(* Logix 5000 AddOnInstructionDefinition export SetupSignVariables; software revision 17.00 *)

ADD_ON_INSTRUCTION SetupSignVariables   (* revision 1.0, vendor Electronic Displays, Inc., ExecuteEnableInFalse *)
// Setup to
// Four Variables
// to LED Sign
// Revision note:
// Original Release
// 11-01-2012
// c.elston
VAR_IN_OUT
   Address : STRING; {required}   // "00" = all signs "01" = address 01 "02" = address 02 etc...(see protocol)
   FileLabel : STRING; {required}   // "A" = default etc...(see protocol)
END_VAR
VAR_INPUT
   ENVariable1Message : BOOL; {visible}   // 0 = don't setup variable 1 = setup variable
END_VAR
VAR_IN_OUT
   Variable1Name : STRING; {required}   // Name of variable Default is = U
END_VAR
VAR_INPUT
   ENVariable2Message : BOOL; {visible}   // 0 = don't setup variable 1 = setup variable
END_VAR
VAR_IN_OUT
   Variable2Name : STRING; {required}   // Name of variable Default is = V
END_VAR
VAR_INPUT
   ENVariable3Message : BOOL; {visible}   // 0 = don't setup variable 1 = setup variable
END_VAR
VAR_IN_OUT
   Variable3Name : STRING; {required}   // Name of variable Default is = W
END_VAR
VAR_INPUT
   ENVariable4Message : BOOL; {visible}   // 0 = don't setup variable 1 = setup variable
END_VAR
VAR_IN_OUT
   Variable4Name : STRING; {required}   // Name of variable Default is = X
END_VAR
VAR_OUTPUT
   EN : BOOL; {visible}   // Instruction Interface Enable Bit
   DN : BOOL; {visible}   // Instruction Interface Done Bit
   ER : BOOL; {visible}   // Instruction Interface Error Bit
   IP : BOOL; {visible}   // Instruction Interface InProcess Bit
END_VAR
VAR_IN_OUT
   map_SignInput : SINT[32]; {required}   // Ethernet/IP LEDSIGN.I Data I/O Mapping
   map_SignOutput : SINT[496]; {required}   // Ethernet/IP LEDSIGN.O Data I/O Mapping
   Packet1Sent : STRING; {required}   // The actual packet sent to the sign (Packet1)
   Packet2Sent : STRING; {required}   // The actual packet sent to the sign (Packet2)
   Packet3Sent : STRING; {required}   // The actual packet sent to the sign (Packet3)
END_VAR
VAR
   SEQ : DINT;   // Sequence Number
   OktoCycle : BOOL;   // Ok to Cycle
   InCycle : BOOL;   // Incycle
   Error : BOOL;   // Error
   Enabled : BOOL;   // Enable ON Bit
   Done : BOOL;   // Done
   Disabled : BOOL;   // Disabled OFF Bit
   SignETX : STRING := '^C';   // DO NOT EDIT = ^C
   SignFileLabel : STRING;
   SignSOH : STRING := '^A';   // DO NOT EDIT = ^A
   SignAddress : STRING;
   SignSTX : STRING := '^B';   // DO NOT EDIT = ^B
   SignNULL : STRING;
   SignVariable4 : STRING;
   SignVariable3 : STRING;
   SignVariable2 : STRING;
   SignVariable1 : STRING;
   SignSetMemoryCommand : STRING := 'SM';   // DO NOT EDIT = SM
   SignCommandCode : STRING := 'C';   // DO NOT EDIT = C
   SignSizeVariableCommand : STRING := '0010';   // DO NOT EDIT = 0010 (16 bytes of memory) enough for 16 characters
   SignFileVariableCommand : STRING := 'V';   // DO NOT EDIT = V
   TotalPacketCount : DINT[7];   // Total Character Count
   Select : DINT;   // Packet Array Select
   PacketMax : DINT := 82;   // Max Packet Count
   PacketCount : DINT[7];
   Packet6Offset : DINT;
   Packet5Offset : DINT;
   Packet4Offset : DINT;
   Packet3Offset : DINT;
   Packet2Offset : DINT;
   Packet1Offset : DINT;
   Packet : STRING[7];   // Packet Array to send to sign
END_VAR

ROUTINE EnableInFalse   (* ladder *)
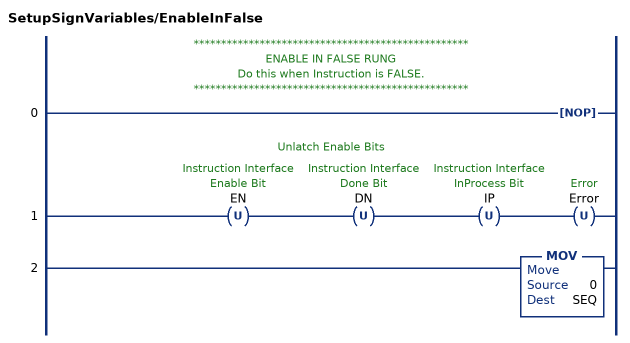
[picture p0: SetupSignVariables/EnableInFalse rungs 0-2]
   // **************************************************
   // ENABLE IN FALSE RUNG
   // Do this when Instruction is FALSE.
   // **************************************************
   0: NOP();
   // Unlatch Enable Bits
   1: OTU(EN)OTU(DN)OTU(IP)OTU(Error);
   2: MOV(0,SEQ);
END_ROUTINE

ROUTINE Logic   (* ladder *)
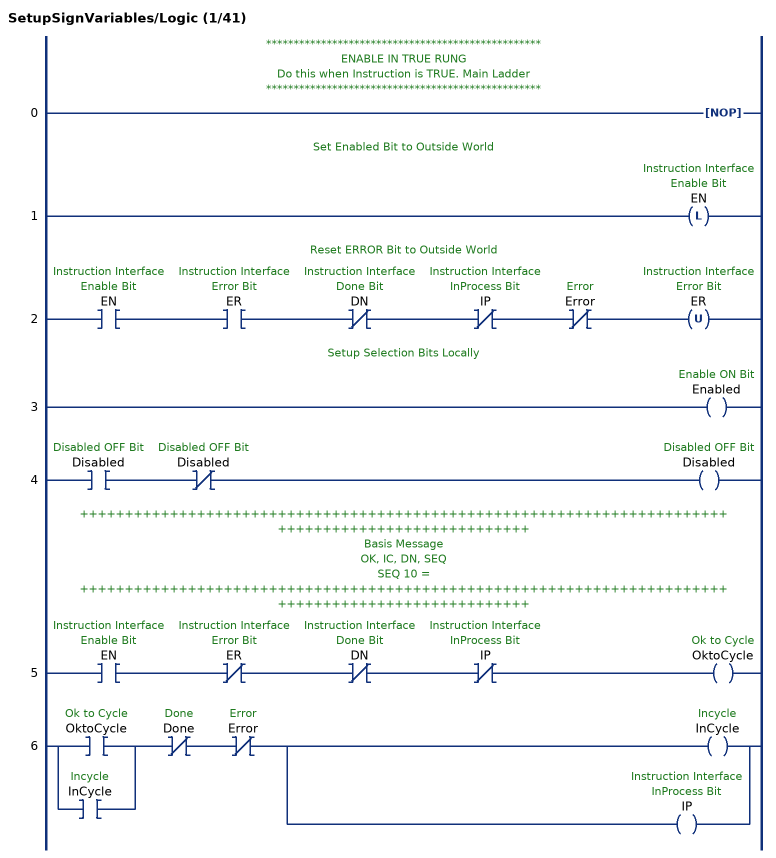
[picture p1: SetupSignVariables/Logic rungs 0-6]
   // **************************************************
   // ENABLE IN TRUE RUNG
   // Do this when Instruction is TRUE. Main Ladder
   // **************************************************
   0: NOP();
   // Set Enabled Bit to Outside World
   1: OTL(EN);
   // Reset ERROR Bit to Outside World
   2: XIC(EN)XIC(ER)XIO(DN)XIO(IP)XIO(Error)OTU(ER);
   // Setup Selection Bits Locally
   3: OTE(Enabled);
   4: XIC(Disabled)XIO(Disabled)OTE(Disabled);
   // ++++++++++++++++++++++++++++++++++++++++++++++++++++++++++++++++++++++++++++++++++++++++++++++++++++
   // Basis Message
   // OK, IC, DN, SEQ
   // SEQ 10 =
   // ++++++++++++++++++++++++++++++++++++++++++++++++++++++++++++++++++++++++++++++++++++++++++++++++++++
   5: XIC(EN)XIO(ER)XIO(DN)XIO(IP)OTE(OktoCycle);
   6: [XIC(OktoCycle) ,XIC(InCycle) ]XIO(Done)XIO(Error)[OTE(InCycle) ,OTE(IP) ];
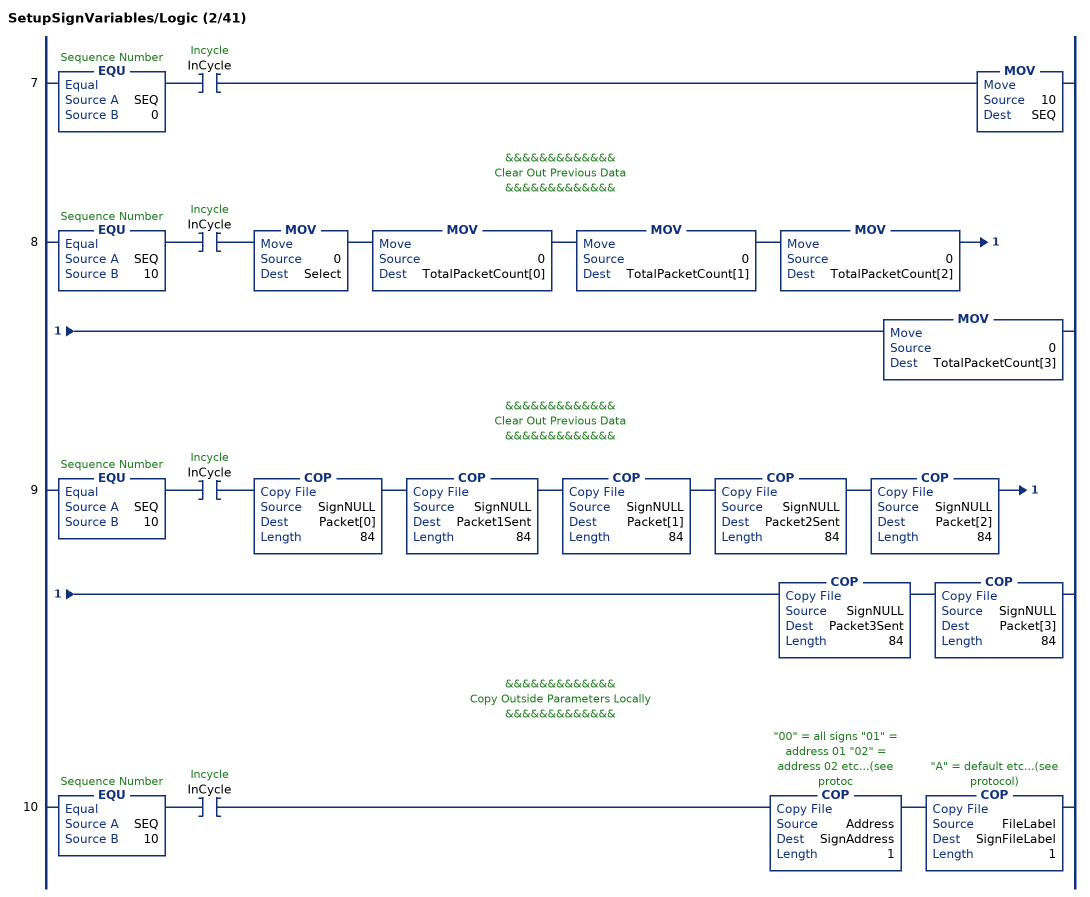
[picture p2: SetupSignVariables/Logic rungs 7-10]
   7: EQU(SEQ,0)XIC(InCycle)MOV(10,SEQ);
   // &&&&&&&&&&&&&
   // Clear Out Previous Data
   // &&&&&&&&&&&&&
   8: EQU(SEQ,10)XIC(InCycle)MOV(0,Select)MOV(0,TotalPacketCount[0])MOV(0,TotalPacketCount[1])MOV(0,TotalPacketCount[2])MOV(0,TotalPacketCount[3]);
   // &&&&&&&&&&&&&
   // Clear Out Previous Data
   // &&&&&&&&&&&&&
   9: EQU(SEQ,10)XIC(InCycle)COP(SignNULL,Packet[0],84)COP(SignNULL,Packet1Sent,84)COP(SignNULL,Packet[1],84)COP(SignNULL,Packet2Sent,84)COP(SignNULL,Packet[2],84)COP(SignNULL,Packet3Sent,84)COP(SignNULL,Packet[3],84);
   // &&&&&&&&&&&&&
   // Copy Outside Parameters Locally
   // &&&&&&&&&&&&&
   10: EQU(SEQ,10)XIC(InCycle)COP(Address,SignAddress,1)COP(FileLabel,SignFileLabel,1);
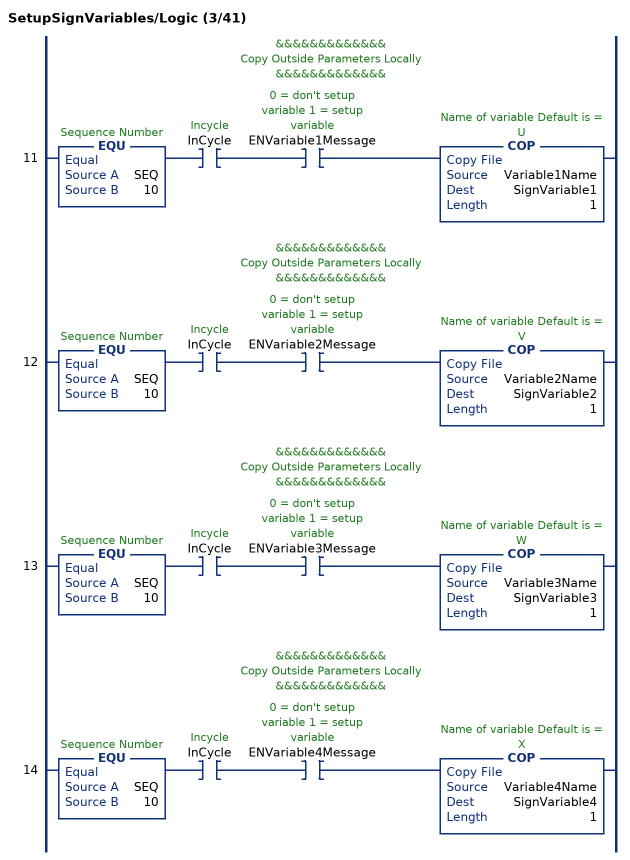
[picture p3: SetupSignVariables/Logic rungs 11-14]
   // &&&&&&&&&&&&&
   // Copy Outside Parameters Locally
   // &&&&&&&&&&&&&
   11: EQU(SEQ,10)XIC(InCycle)XIC(ENVariable1Message)COP(Variable1Name,SignVariable1,1);
   // &&&&&&&&&&&&&
   // Copy Outside Parameters Locally
   // &&&&&&&&&&&&&
   12: EQU(SEQ,10)XIC(InCycle)XIC(ENVariable2Message)COP(Variable2Name,SignVariable2,1);
   // &&&&&&&&&&&&&
   // Copy Outside Parameters Locally
   // &&&&&&&&&&&&&
   13: EQU(SEQ,10)XIC(InCycle)XIC(ENVariable3Message)COP(Variable3Name,SignVariable3,1);
   // &&&&&&&&&&&&&
   // Copy Outside Parameters Locally
   // &&&&&&&&&&&&&
   14: EQU(SEQ,10)XIC(InCycle)XIC(ENVariable4Message)COP(Variable4Name,SignVariable4,1);
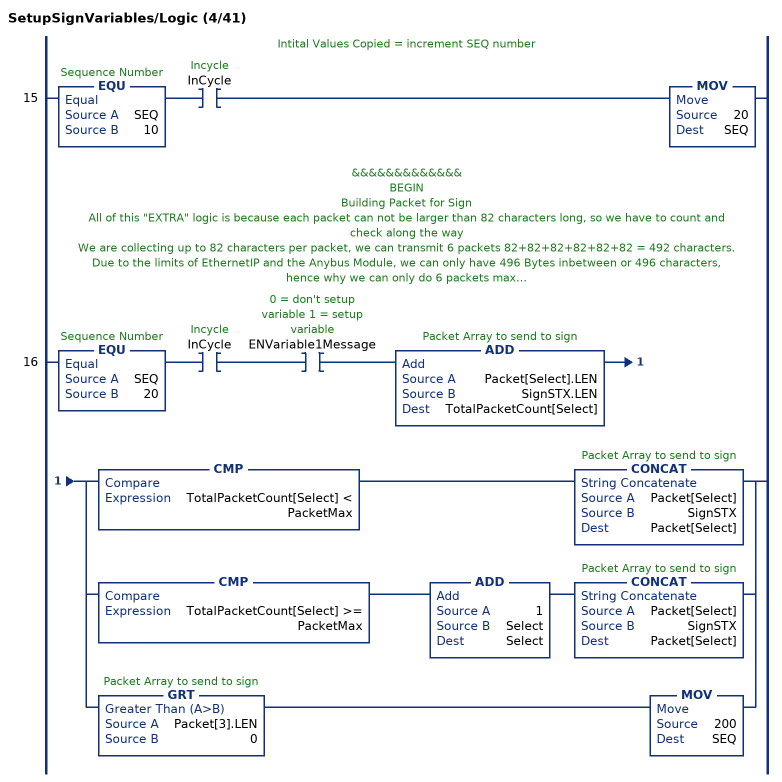
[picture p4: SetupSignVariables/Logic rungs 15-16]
   // Intital Values Copied = increment SEQ number
   15: EQU(SEQ,10)XIC(InCycle)MOV(20,SEQ);
   // &&&&&&&&&&&&&
   // BEGIN
   // Building Packet for Sign
   // All of this "EXTRA" logic is because each packet can not be larger than 82 characters long, so we have to count and check along the way
   // We are collecting up to 82 characters per packet, we can transmit 6 packets 82+82+82+82+82+82 = 492 characters.
   // Due to the limits of EthernetIP and the Anybus Module, we can only have 496 Bytes inbetween or 496 characters, hence why we can only do 6 packets max.
   // Once we exceed this, we will fault and ERROR trap any windy typing people.
   // In this instruction below, it's so small, we are only using 3 packets max.
   // &&&&&&&&&&&&&
   16: EQU(SEQ,20)XIC(InCycle)XIC(ENVariable1Message)ADD(Packet[Select].LEN,SignSTX.LEN,TotalPacketCount[Select])[CMP(TotalPacketCount[Select] < PacketMax) CONCAT(Packet[Select],SignSTX,Packet[Select]) ,CMP(TotalPacketCount[Select] >= PacketMax) ADD(1,Select,Select) CONCAT(Packet[Select],SignSTX,Packet[Select]) ,GRT(Packet[3].LEN,0) MOV(200,SEQ) ];
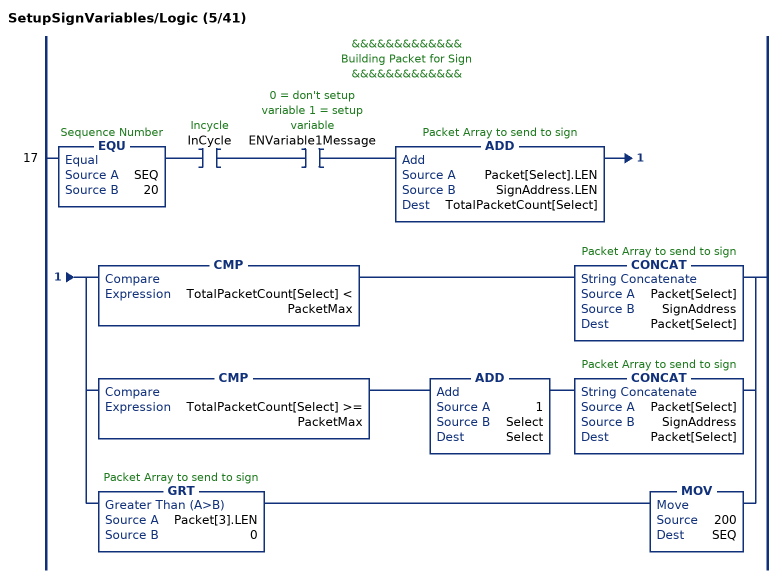
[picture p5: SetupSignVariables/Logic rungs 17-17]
   // &&&&&&&&&&&&&
   // Building Packet for Sign
   // &&&&&&&&&&&&&
   17: EQU(SEQ,20)XIC(InCycle)XIC(ENVariable1Message)ADD(Packet[Select].LEN,SignAddress.LEN,TotalPacketCount[Select])[CMP(TotalPacketCount[Select] < PacketMax) CONCAT(Packet[Select],SignAddress,Packet[Select]) ,CMP(TotalPacketCount[Select] >= PacketMax) ADD(1,Select,Select) CONCAT(Packet[Select],SignAddress,Packet[Select]) ,GRT(Packet[3].LEN,0) MOV(200,SEQ) ];
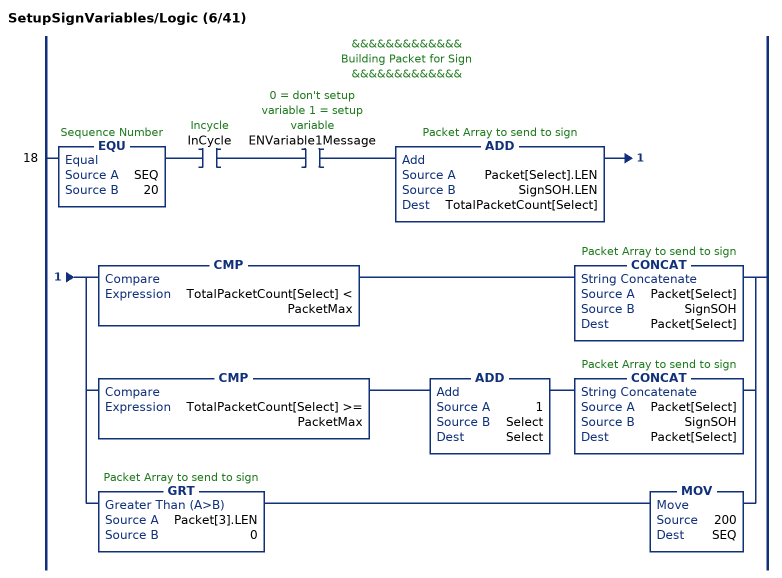
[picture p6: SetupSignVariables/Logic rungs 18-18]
   // &&&&&&&&&&&&&
   // Building Packet for Sign
   // &&&&&&&&&&&&&
   18: EQU(SEQ,20)XIC(InCycle)XIC(ENVariable1Message)ADD(Packet[Select].LEN,SignSOH.LEN,TotalPacketCount[Select])[CMP(TotalPacketCount[Select] < PacketMax) CONCAT(Packet[Select],SignSOH,Packet[Select]) ,CMP(TotalPacketCount[Select] >= PacketMax) ADD(1,Select,Select) CONCAT(Packet[Select],SignSOH,Packet[Select]) ,GRT(Packet[3].LEN,0) MOV(200,SEQ) ];
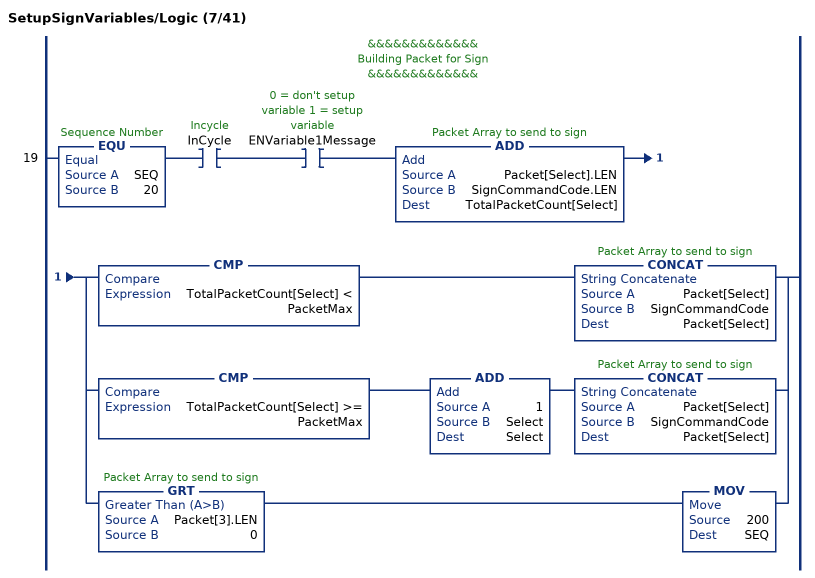
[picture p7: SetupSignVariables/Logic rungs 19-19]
   // &&&&&&&&&&&&&
   // Building Packet for Sign
   // &&&&&&&&&&&&&
   19: EQU(SEQ,20)XIC(InCycle)XIC(ENVariable1Message)ADD(Packet[Select].LEN,SignCommandCode.LEN,TotalPacketCount[Select])[CMP(TotalPacketCount[Select] < PacketMax) CONCAT(Packet[Select],SignCommandCode,Packet[Select]) ,CMP(TotalPacketCount[Select] >= PacketMax) ADD(1,Select,Select) CONCAT(Packet[Select],SignCommandCode,Packet[Select]) ,GRT(Packet[3].LEN,0) MOV(200,SEQ) ];
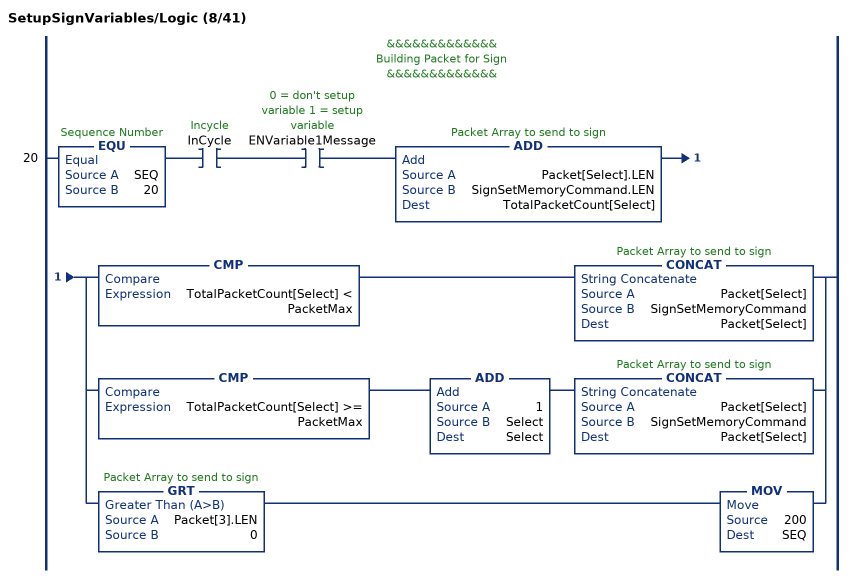
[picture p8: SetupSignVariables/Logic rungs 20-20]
   // &&&&&&&&&&&&&
   // Building Packet for Sign
   // &&&&&&&&&&&&&
   20: EQU(SEQ,20)XIC(InCycle)XIC(ENVariable1Message)ADD(Packet[Select].LEN,SignSetMemoryCommand.LEN,TotalPacketCount[Select])[CMP(TotalPacketCount[Select] < PacketMax) CONCAT(Packet[Select],SignSetMemoryCommand,Packet[Select]) ,CMP(TotalPacketCount[Select] >= PacketMax) ADD(1,Select,Select) CONCAT(Packet[Select],SignSetMemoryCommand,Packet[Select]) ,GRT(Packet[3].LEN,0) MOV(200,SEQ) ];
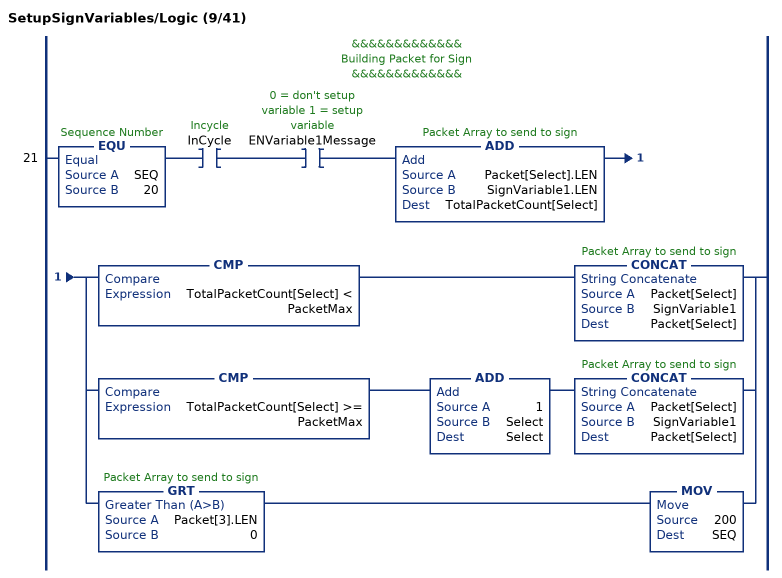
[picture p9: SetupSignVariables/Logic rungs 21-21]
   // &&&&&&&&&&&&&
   // Building Packet for Sign
   // &&&&&&&&&&&&&
   21: EQU(SEQ,20)XIC(InCycle)XIC(ENVariable1Message)ADD(Packet[Select].LEN,SignVariable1.LEN,TotalPacketCount[Select])[CMP(TotalPacketCount[Select] < PacketMax) CONCAT(Packet[Select],SignVariable1,Packet[Select]) ,CMP(TotalPacketCount[Select] >= PacketMax) ADD(1,Select,Select) CONCAT(Packet[Select],SignVariable1,Packet[Select]) ,GRT(Packet[3].LEN,0) MOV(200,SEQ) ];
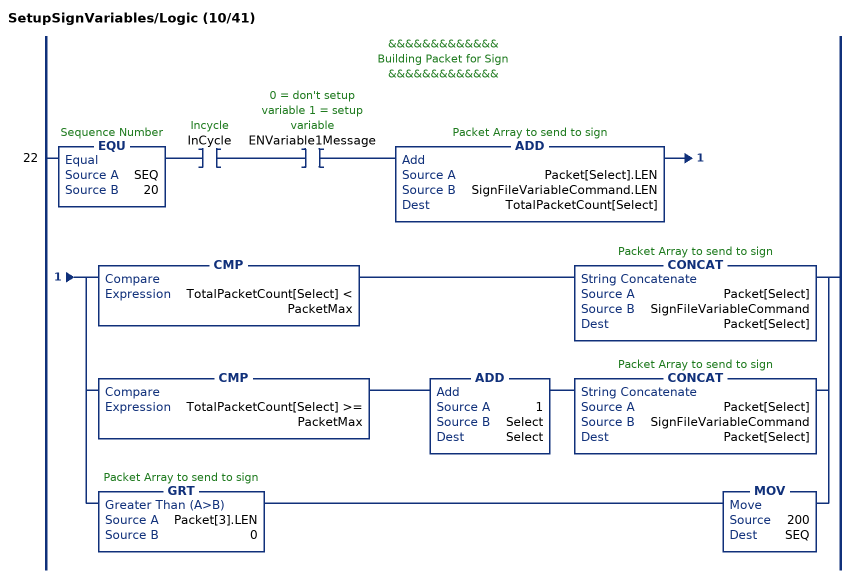
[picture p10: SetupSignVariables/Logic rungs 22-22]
   // &&&&&&&&&&&&&
   // Building Packet for Sign
   // &&&&&&&&&&&&&
   22: EQU(SEQ,20)XIC(InCycle)XIC(ENVariable1Message)ADD(Packet[Select].LEN,SignFileVariableCommand.LEN,TotalPacketCount[Select])[CMP(TotalPacketCount[Select] < PacketMax) CONCAT(Packet[Select],SignFileVariableCommand,Packet[Select]) ,CMP(TotalPacketCount[Select] >= PacketMax) ADD(1,Select,Select) CONCAT(Packet[Select],SignFileVariableCommand,Packet[Select]) ,GRT(Packet[3].LEN,0) MOV(200,SEQ) ];
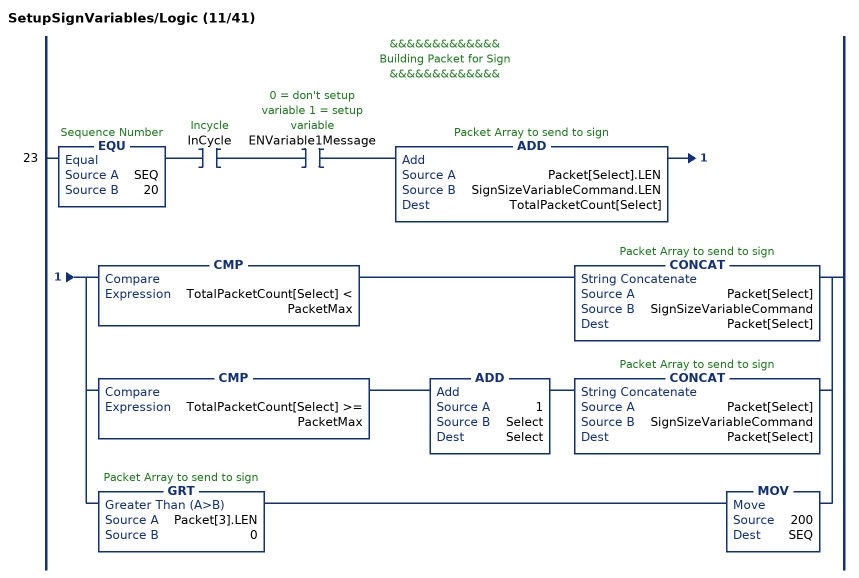
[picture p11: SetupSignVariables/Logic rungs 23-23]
   // &&&&&&&&&&&&&
   // Building Packet for Sign
   // &&&&&&&&&&&&&
   23: EQU(SEQ,20)XIC(InCycle)XIC(ENVariable1Message)ADD(Packet[Select].LEN,SignSizeVariableCommand.LEN,TotalPacketCount[Select])[CMP(TotalPacketCount[Select] < PacketMax) CONCAT(Packet[Select],SignSizeVariableCommand,Packet[Select]) ,CMP(TotalPacketCount[Select] >= PacketMax) ADD(1,Select,Select) CONCAT(Packet[Select],SignSizeVariableCommand,Packet[Select]) ,GRT(Packet[3].LEN,0) MOV(200,SEQ) ];
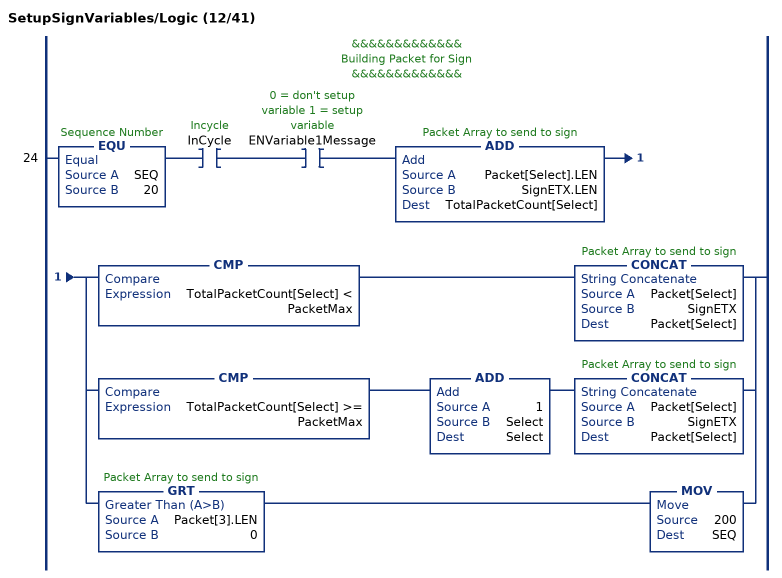
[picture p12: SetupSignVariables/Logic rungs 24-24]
   // &&&&&&&&&&&&&
   // Building Packet for Sign
   // &&&&&&&&&&&&&
   24: EQU(SEQ,20)XIC(InCycle)XIC(ENVariable1Message)ADD(Packet[Select].LEN,SignETX.LEN,TotalPacketCount[Select])[CMP(TotalPacketCount[Select] < PacketMax) CONCAT(Packet[Select],SignETX,Packet[Select]) ,CMP(TotalPacketCount[Select] >= PacketMax) ADD(1,Select,Select) CONCAT(Packet[Select],SignETX,Packet[Select]) ,GRT(Packet[3].LEN,0) MOV(200,SEQ) ];
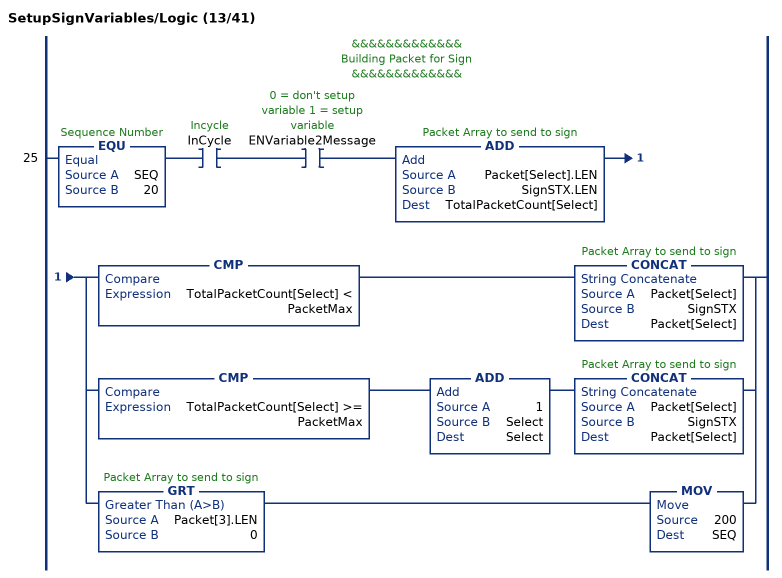
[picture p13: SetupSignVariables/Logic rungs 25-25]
   // &&&&&&&&&&&&&
   // Building Packet for Sign
   // &&&&&&&&&&&&&
   25: EQU(SEQ,20)XIC(InCycle)XIC(ENVariable2Message)ADD(Packet[Select].LEN,SignSTX.LEN,TotalPacketCount[Select])[CMP(TotalPacketCount[Select] < PacketMax) CONCAT(Packet[Select],SignSTX,Packet[Select]) ,CMP(TotalPacketCount[Select] >= PacketMax) ADD(1,Select,Select) CONCAT(Packet[Select],SignSTX,Packet[Select]) ,GRT(Packet[3].LEN,0) MOV(200,SEQ) ];
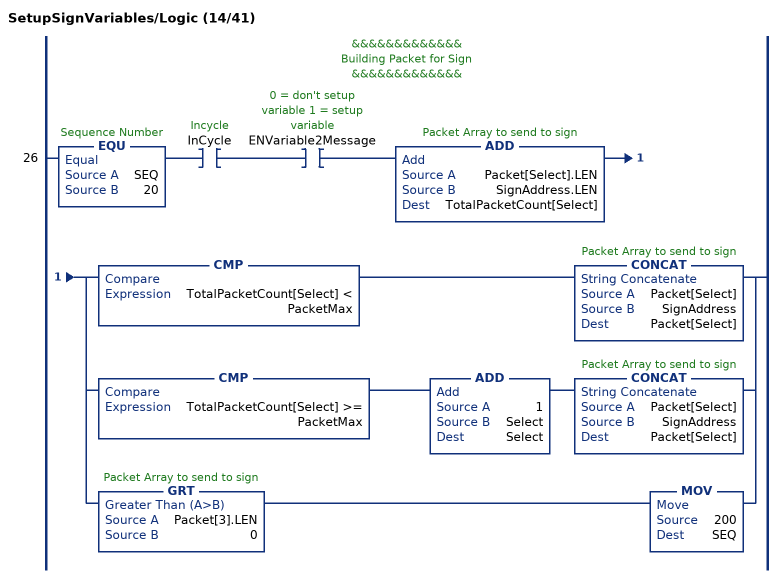
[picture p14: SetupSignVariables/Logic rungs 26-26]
   // &&&&&&&&&&&&&
   // Building Packet for Sign
   // &&&&&&&&&&&&&
   26: EQU(SEQ,20)XIC(InCycle)XIC(ENVariable2Message)ADD(Packet[Select].LEN,SignAddress.LEN,TotalPacketCount[Select])[CMP(TotalPacketCount[Select] < PacketMax) CONCAT(Packet[Select],SignAddress,Packet[Select]) ,CMP(TotalPacketCount[Select] >= PacketMax) ADD(1,Select,Select) CONCAT(Packet[Select],SignAddress,Packet[Select]) ,GRT(Packet[3].LEN,0) MOV(200,SEQ) ];
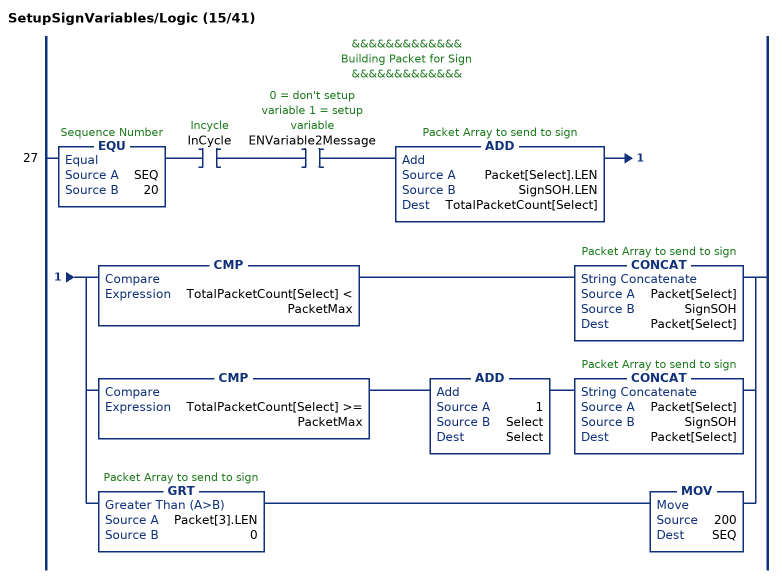
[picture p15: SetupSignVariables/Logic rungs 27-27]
   // &&&&&&&&&&&&&
   // Building Packet for Sign
   // &&&&&&&&&&&&&
   27: EQU(SEQ,20)XIC(InCycle)XIC(ENVariable2Message)ADD(Packet[Select].LEN,SignSOH.LEN,TotalPacketCount[Select])[CMP(TotalPacketCount[Select] < PacketMax) CONCAT(Packet[Select],SignSOH,Packet[Select]) ,CMP(TotalPacketCount[Select] >= PacketMax) ADD(1,Select,Select) CONCAT(Packet[Select],SignSOH,Packet[Select]) ,GRT(Packet[3].LEN,0) MOV(200,SEQ) ];
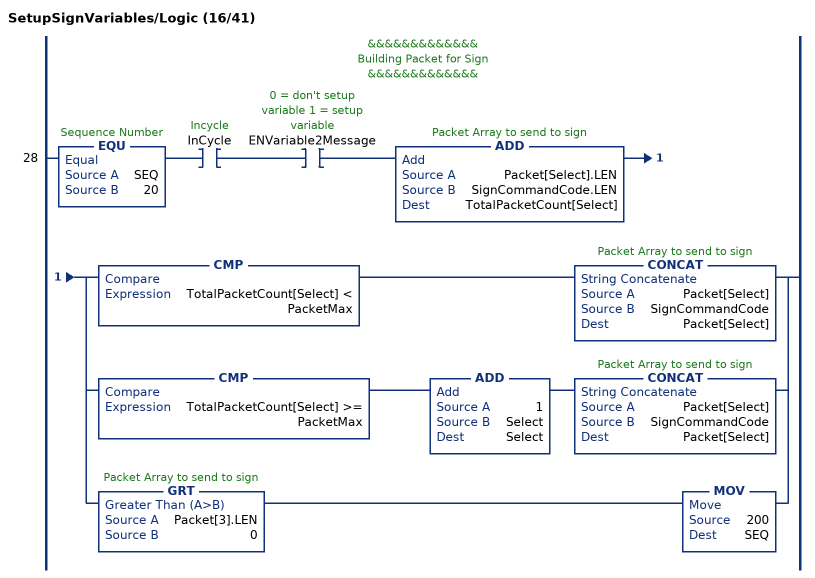
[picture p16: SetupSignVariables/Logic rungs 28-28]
   // &&&&&&&&&&&&&
   // Building Packet for Sign
   // &&&&&&&&&&&&&
   28: EQU(SEQ,20)XIC(InCycle)XIC(ENVariable2Message)ADD(Packet[Select].LEN,SignCommandCode.LEN,TotalPacketCount[Select])[CMP(TotalPacketCount[Select] < PacketMax) CONCAT(Packet[Select],SignCommandCode,Packet[Select]) ,CMP(TotalPacketCount[Select] >= PacketMax) ADD(1,Select,Select) CONCAT(Packet[Select],SignCommandCode,Packet[Select]) ,GRT(Packet[3].LEN,0) MOV(200,SEQ) ];
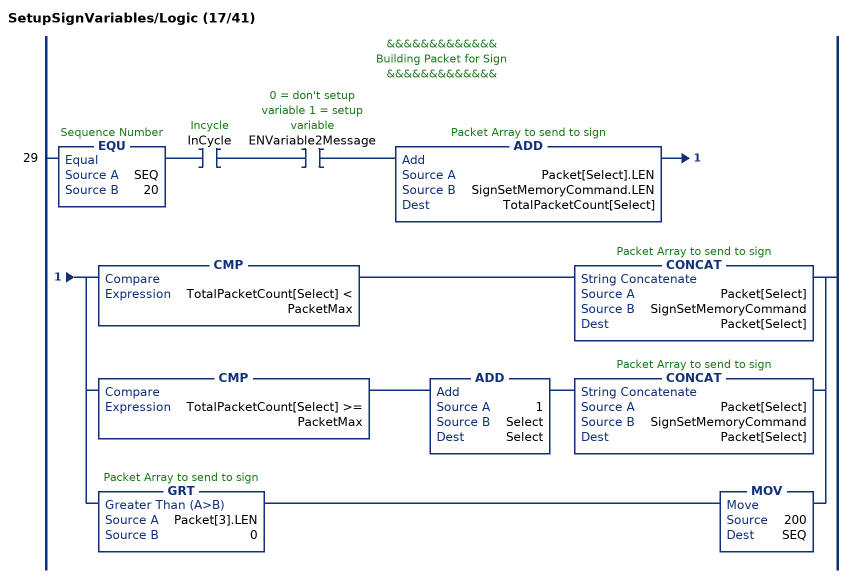
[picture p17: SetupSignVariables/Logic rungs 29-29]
   // &&&&&&&&&&&&&
   // Building Packet for Sign
   // &&&&&&&&&&&&&
   29: EQU(SEQ,20)XIC(InCycle)XIC(ENVariable2Message)ADD(Packet[Select].LEN,SignSetMemoryCommand.LEN,TotalPacketCount[Select])[CMP(TotalPacketCount[Select] < PacketMax) CONCAT(Packet[Select],SignSetMemoryCommand,Packet[Select]) ,CMP(TotalPacketCount[Select] >= PacketMax) ADD(1,Select,Select) CONCAT(Packet[Select],SignSetMemoryCommand,Packet[Select]) ,GRT(Packet[3].LEN,0) MOV(200,SEQ) ];
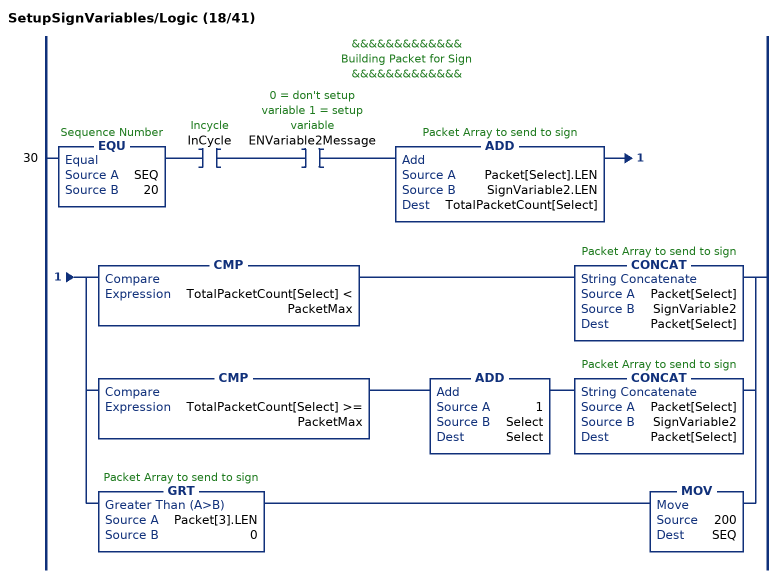
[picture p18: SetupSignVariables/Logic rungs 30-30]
   // &&&&&&&&&&&&&
   // Building Packet for Sign
   // &&&&&&&&&&&&&
   30: EQU(SEQ,20)XIC(InCycle)XIC(ENVariable2Message)ADD(Packet[Select].LEN,SignVariable2.LEN,TotalPacketCount[Select])[CMP(TotalPacketCount[Select] < PacketMax) CONCAT(Packet[Select],SignVariable2,Packet[Select]) ,CMP(TotalPacketCount[Select] >= PacketMax) ADD(1,Select,Select) CONCAT(Packet[Select],SignVariable2,Packet[Select]) ,GRT(Packet[3].LEN,0) MOV(200,SEQ) ];
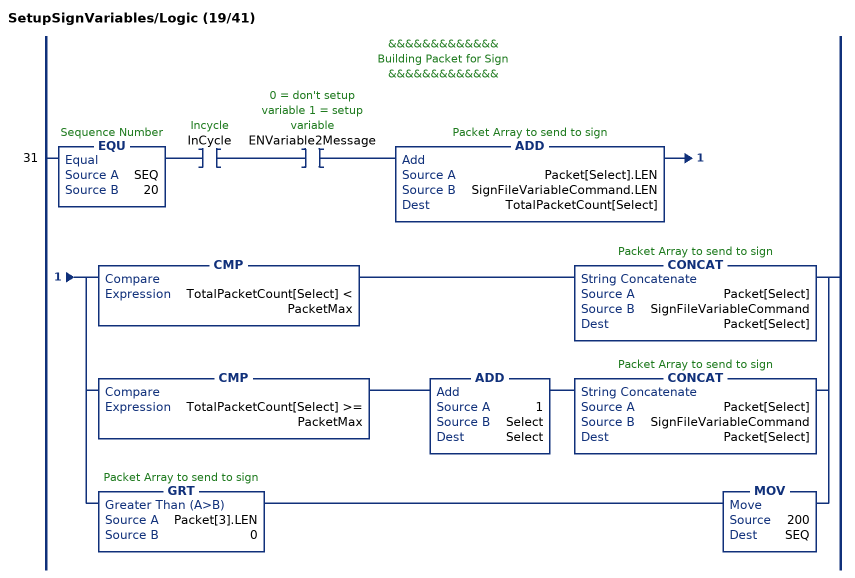
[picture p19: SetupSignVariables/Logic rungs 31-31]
   // &&&&&&&&&&&&&
   // Building Packet for Sign
   // &&&&&&&&&&&&&
   31: EQU(SEQ,20)XIC(InCycle)XIC(ENVariable2Message)ADD(Packet[Select].LEN,SignFileVariableCommand.LEN,TotalPacketCount[Select])[CMP(TotalPacketCount[Select] < PacketMax) CONCAT(Packet[Select],SignFileVariableCommand,Packet[Select]) ,CMP(TotalPacketCount[Select] >= PacketMax) ADD(1,Select,Select) CONCAT(Packet[Select],SignFileVariableCommand,Packet[Select]) ,GRT(Packet[3].LEN,0) MOV(200,SEQ) ];
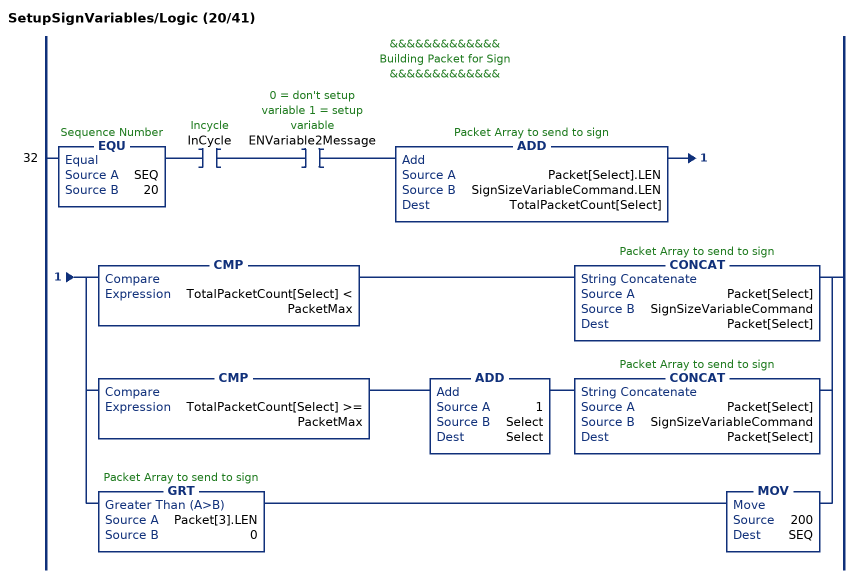
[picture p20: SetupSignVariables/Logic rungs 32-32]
   // &&&&&&&&&&&&&
   // Building Packet for Sign
   // &&&&&&&&&&&&&
   32: EQU(SEQ,20)XIC(InCycle)XIC(ENVariable2Message)ADD(Packet[Select].LEN,SignSizeVariableCommand.LEN,TotalPacketCount[Select])[CMP(TotalPacketCount[Select] < PacketMax) CONCAT(Packet[Select],SignSizeVariableCommand,Packet[Select]) ,CMP(TotalPacketCount[Select] >= PacketMax) ADD(1,Select,Select) CONCAT(Packet[Select],SignSizeVariableCommand,Packet[Select]) ,GRT(Packet[3].LEN,0) MOV(200,SEQ) ];
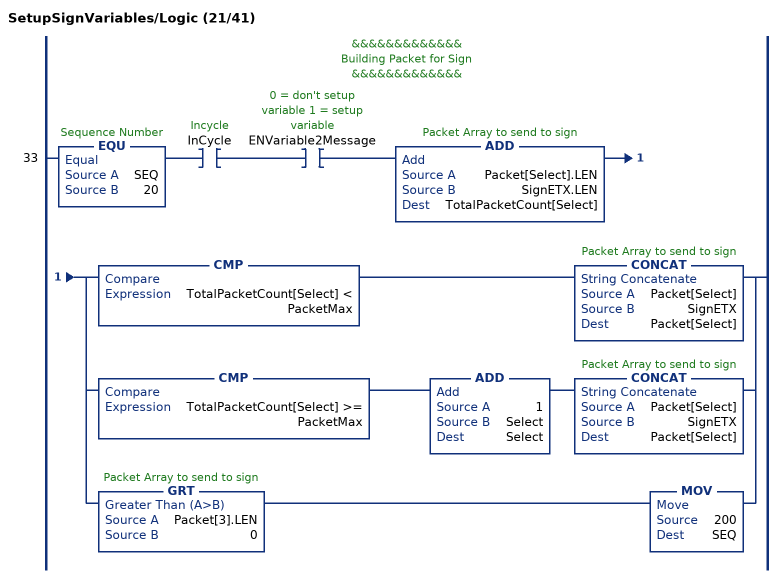
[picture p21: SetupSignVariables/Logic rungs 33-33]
   // &&&&&&&&&&&&&
   // Building Packet for Sign
   // &&&&&&&&&&&&&
   33: EQU(SEQ,20)XIC(InCycle)XIC(ENVariable2Message)ADD(Packet[Select].LEN,SignETX.LEN,TotalPacketCount[Select])[CMP(TotalPacketCount[Select] < PacketMax) CONCAT(Packet[Select],SignETX,Packet[Select]) ,CMP(TotalPacketCount[Select] >= PacketMax) ADD(1,Select,Select) CONCAT(Packet[Select],SignETX,Packet[Select]) ,GRT(Packet[3].LEN,0) MOV(200,SEQ) ];
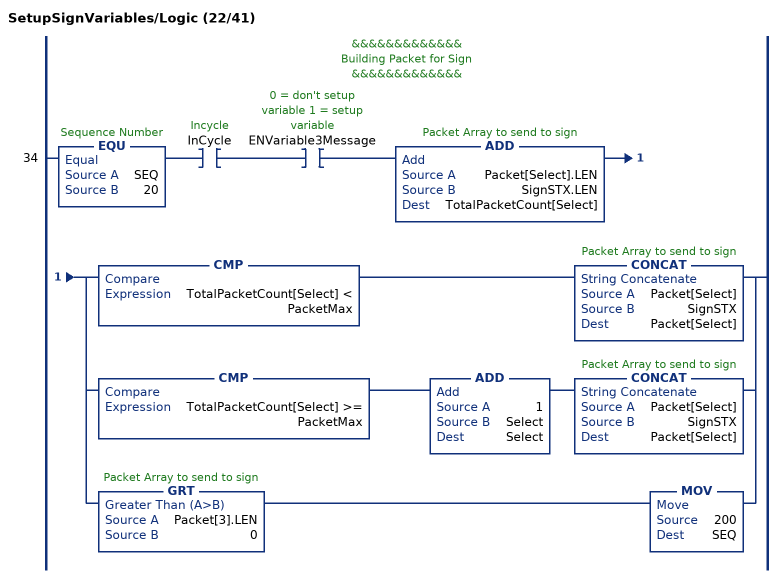
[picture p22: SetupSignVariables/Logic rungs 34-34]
   // &&&&&&&&&&&&&
   // Building Packet for Sign
   // &&&&&&&&&&&&&
   34: EQU(SEQ,20)XIC(InCycle)XIC(ENVariable3Message)ADD(Packet[Select].LEN,SignSTX.LEN,TotalPacketCount[Select])[CMP(TotalPacketCount[Select] < PacketMax) CONCAT(Packet[Select],SignSTX,Packet[Select]) ,CMP(TotalPacketCount[Select] >= PacketMax) ADD(1,Select,Select) CONCAT(Packet[Select],SignSTX,Packet[Select]) ,GRT(Packet[3].LEN,0) MOV(200,SEQ) ];
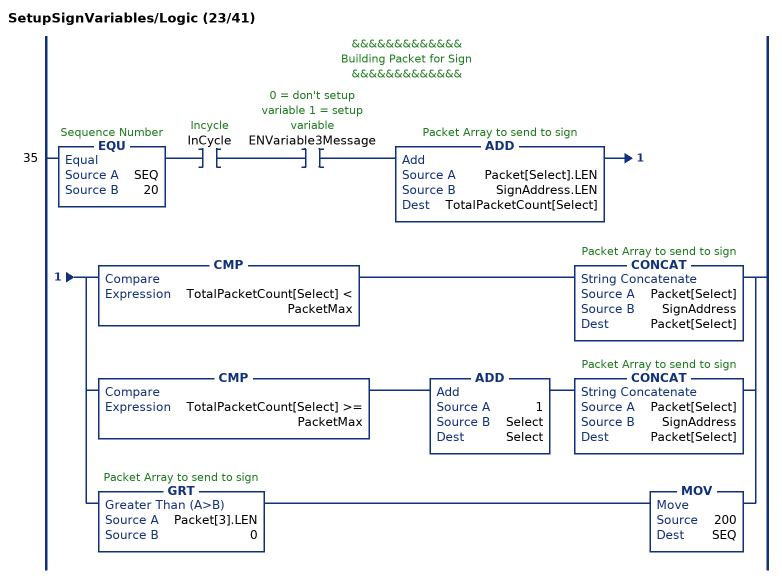
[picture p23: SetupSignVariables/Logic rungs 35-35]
   // &&&&&&&&&&&&&
   // Building Packet for Sign
   // &&&&&&&&&&&&&
   35: EQU(SEQ,20)XIC(InCycle)XIC(ENVariable3Message)ADD(Packet[Select].LEN,SignAddress.LEN,TotalPacketCount[Select])[CMP(TotalPacketCount[Select] < PacketMax) CONCAT(Packet[Select],SignAddress,Packet[Select]) ,CMP(TotalPacketCount[Select] >= PacketMax) ADD(1,Select,Select) CONCAT(Packet[Select],SignAddress,Packet[Select]) ,GRT(Packet[3].LEN,0) MOV(200,SEQ) ];
